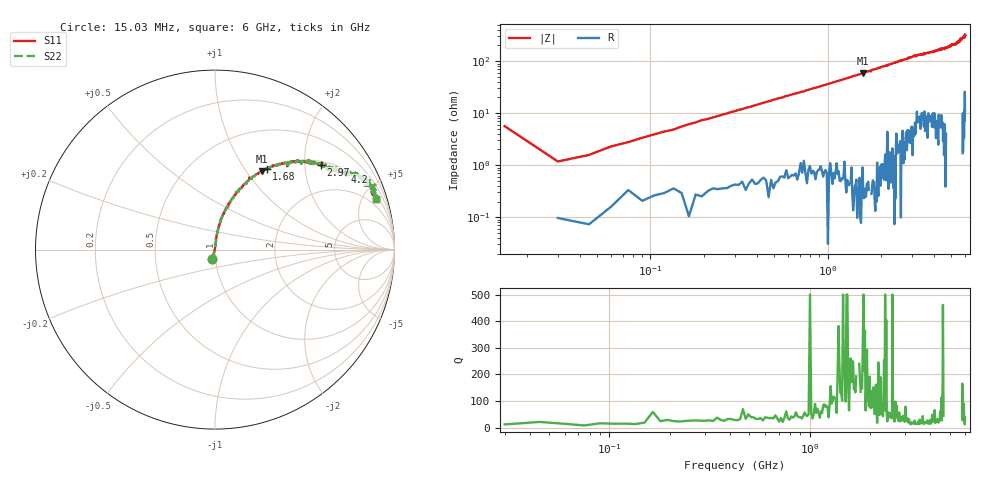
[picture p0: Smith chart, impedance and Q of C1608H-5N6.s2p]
!	Network	Analyzer	HP8753E.07.74:	Oct	30	2002	Serial	No.	JP38451487
!	Hewlett-Packard
!	7	Sep	2009	10:13:04
!	Frequency	S11	S21	S12	S22
#	HZ	S	RI	R	50
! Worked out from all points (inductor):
!   400 points, 15.03 MHz to 6 GHz, reference 50 ohm
!   read as one part in series: L = 5.83 nH near 45.03 MHz
!   highest Q = 247 at 1.59 GHz (marker M1), where L = 5.92 nH
!   S11 on the Smith chart (normalised r, x): 15.03 MHz: 0.96, -0.11; 1.68 GHz: 1.01, +1.26; 2.97 GHz: 1.09, +2.40; 4.2 GHz: 1.09, +3.28; 6 GHz: 1.33, +6.25
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1.502992e7  -0.0152 -0.0545  1.02 0.0545  1.02 0.0545  -0.0152 -0.0545
3.002985e7  0.0012 0.0117  0.999 -0.0117  0.999 -0.0117  0.0012 0.0117
6.00297e7  0.00222 0.0228  0.998 -0.0228  0.998 -0.0228  0.00222 0.0228
1.200294e8  0.00471 0.044  0.995 -0.044  0.995 -0.044  0.00471 0.044
1.95029e8  0.0076 0.0725  0.992 -0.0725  0.992 -0.0725  0.0076 0.0725
2.850286e8  0.0145 0.103  0.985 -0.103  0.985 -0.103  0.0145 0.103
5.850271e8  0.0509 0.202  0.949 -0.202  0.949 -0.202  0.0509 0.202
1.020025e9  0.124 0.32  0.876 -0.32  0.876 -0.32  0.124 0.32
1.590022e9  0.26 0.436  0.74 -0.436  0.74 -0.436  0.26 0.436
1.680022e9  0.287 0.449  0.713 -0.449  0.713 -0.449  0.287 0.449
2.01002e9  0.373 0.477  0.627 -0.477  0.627 -0.477  0.373 0.477
2.970015e9  0.588 0.474  0.412 -0.474  0.412 -0.474  0.588 0.474
3.015015e9  0.598 0.484  0.402 -0.484  0.402 -0.484  0.598 0.484
4.00501e9  0.706 0.439  0.294 -0.439  0.294 -0.439  0.706 0.439
4.200009e9  0.724 0.433  0.276 -0.433  0.276 -0.433  0.724 0.433
5.010005e9  0.81 0.405  0.19 -0.405  0.19 -0.405  0.81 0.405
5.295004e9  0.822 0.403  0.178 -0.403  0.178 -0.403  0.822 0.403
5.535002e9  0.834 0.357  0.166 -0.357  0.166 -0.357  0.834 0.357
5.565002e9  0.893 0.36  0.107 -0.36  0.107 -0.36  0.893 0.36
5.595002e9  0.855 0.356  0.145 -0.356  0.145 -0.356  0.855 0.356
5.625002e9  0.894 0.332  0.106 -0.332  0.106 -0.332  0.894 0.332
6e9  0.895 0.281  0.105 -0.281  0.105 -0.281  0.895 0.281
